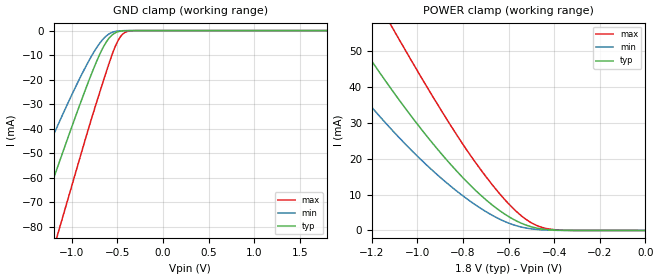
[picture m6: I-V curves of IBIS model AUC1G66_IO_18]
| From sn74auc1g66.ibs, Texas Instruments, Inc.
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[Model]   AUC1G66_IO_18
Model_type  Terminator
| variable   typ   min   max
C_comp   2.86pF   2.61pF   3.02pF
| C_tri-state   2.86pF   2.61pF   3.02pF
[Temperature Range]   40   100   -40
| Ambient temperature   25   85   -40
[Voltage range]   1.8   1.65   1.95
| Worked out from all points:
|   GND clamp passes 1 mA (typ) near -0.53 V on its own axis
|   POWER clamp passes 1 mA (typ) near -0.50 V on its own axis
[GND Clamp]
| AUC1G66_IO_18
|   Voltage   I(typ)   I(min)   I(max)
-2.7V     -221.8mA   -178.5mA   -275mA
-1.675V   -111.5mA   -84.22mA   -148.6mA
-1.63V    -106.7mA   -80.17mA   -143mA
-1.42V    -83.98mA   -61.49mA   -116.7mA
-1.385V   -80.21mA   -58.43mA   -112.3mA
-1.145V   -54.52mA   -37.94mA   -81.86mA
-775mV    -16.85mA   -9.855mA   -34.87mA
-660mV    -7.157mA   -3.626mA   -21.25mA
-570mV    -2.231mA   -936.1uA   -11.07mA
-465mV    -242.2uA   -89.82uA   -2.444mA
-355mV    -11.13uA   -5.239uA   -117.8uA
1.8V      413.4pA    46.18nA    314.7pA
[POWER Clamp]
| AUC1G66_IO_18
|   Voltage   I(typ)   I(min)   I(max)
-2.7V     214.4mA    184.8mA    244.7mA
-1.47V    73.54mA    55.84mA    97.67mA
-1.3V     56.54mA    41.83mA    77.93mA
-1.115V   39.34mA    28.17mA    56.97mA
-1.095V   37.58mA    26.81mA    54.75mA
-930mV    23.98mA    16.46mA    36.95mA
-780mV    13.32mA    8.657mA    22.02mA
-635mV    5.323mA    3.01mA     9.881mA
-535mV    1.766mA    822.1uA    3.615mA
-475mV    637.7uA    272.6uA    1.344mA
-395mV    100.5uA    45.32uA    191.6uA
-35.59fV  413.4pA    716.8pA    379.3pA
